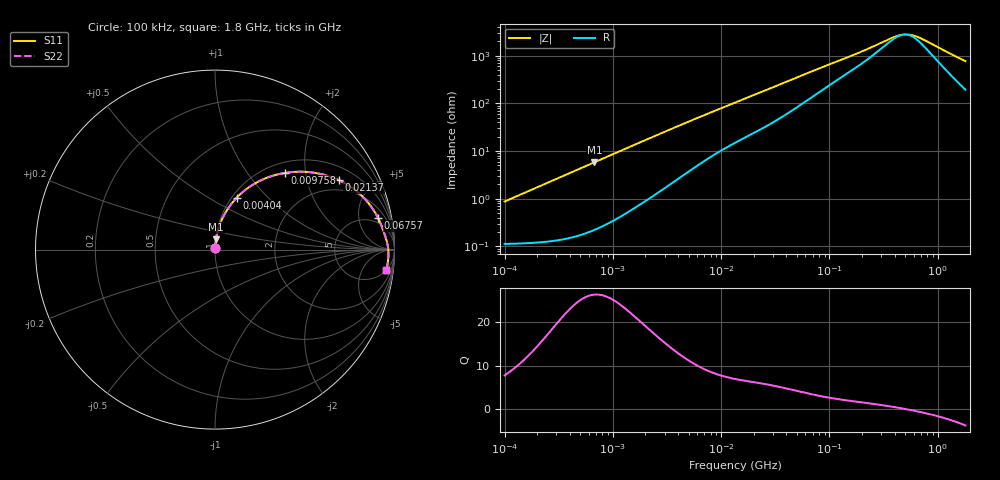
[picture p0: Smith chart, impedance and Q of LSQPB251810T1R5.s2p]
! LSQPB251810T1R5  S-PARAMETER MODEL  ( General Type )
! Model Generated by TAIYO YUDEN Corporation (http://www.ty-top.com)
! Version 2.0
! TAIYO YUDEN Control No. 100810NG22EB-FKC
! Copyright(c) 2009 TAIYO YUDEN CO.,LTD. All Rights Reserved.
! Product Description (link to TY-COMPAS)
! https://ds.yuden.co.jp/TYCOMPAS/or/detail?pn=LSQPB251810T1R5M&u=M
! Products Name : Inductors
! Characteristics :
!  Inductance : 1.5 uH , SRF(min) : 100 MHz , DC Resistance(max) : 0.143 Ohm
!  Rated Current : Saturation :1100 mA , Temp Rise : 1000 mA (40 degC)
!  Case Size : 2.5 x 1.8 / 0.098 x 0.071 [mm/inch] , Thickness : 1.0 / 0.04 [mm/inch]
!  (Conditions: Temperature = 25 degC , DC Bias Current/Voltage = 0A / 0V)
! External Node Assignments :
!  1  o---GGG---o  2
! GND o---------o GND
! Frequency Range : 0.1MHz  -  1800MHz  [ 402 STEP ]
# MHz S RI R 50
! Freq[MHz].  S11 Real  S11 Imag  S21 Real  S21 Imag  S12 Real  S12 Imag  S22 Real  S22 Imag
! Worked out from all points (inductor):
!   401 points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, 100 kHz to 1.8 GHz, reference 50 ohm
!   read as one part in series: L = 1.38 uH near 105 kHz
!   highest Q = 26.4 at 675.7 kHz (marker M1), where L = 1.38 uH
!   self-resonance near 490.3 MHz
!   S11 on the Smith chart (normalised r, x): 100 kHz: 1.00, +0.02; 4.04 MHz: 1.05, +0.67; 9.758 MHz: 1.20, +1.54; 21.37 MHz: 1.52, +3.13; 67.57 MHz: 3.63, +8.90; 1.8 GHz: 5, -15
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0.1  0.0012 0.00865  0.9988 -0.00865  0.9988 -0.00865  0.0012 0.00865
0.516129  0.00374 0.0444  0.9963 -0.0444  0.9963 -0.0444  0.00374 0.0444
0.675738  0.00559 0.0579  0.9944 -0.0579  0.9944 -0.0579  0.00559 0.0579
1.409041  0.0195 0.1179  0.9805 -0.1179  0.9805 -0.1179  0.0195 0.1179
2.66389  0.0601 0.2091  0.9399 -0.2091  0.9399 -0.2091  0.0601 0.2091
4.039851  0.1208 0.289  0.8792 -0.289  0.8792 -0.289  0.1208 0.289
6.126528  0.2245 0.3697  0.7755 -0.3697  0.7755 -0.3697  0.2245 0.3697
9.75753  0.3893 0.4273  0.6107 -0.4273  0.6107 -0.4273  0.3893 0.4273
13.41641  0.5158 0.4324  0.4842 -0.4324  0.4842 -0.4324  0.5158 0.4324
21.36789  0.6882 0.3877  0.3118 -0.3877  0.3118 -0.3877  0.6882 0.3877
27.97575  0.7684 0.341  0.2316 -0.341  0.2316 -0.341  0.7684 0.341
36.62703  0.8296 0.2878  0.1704 -0.2878  0.1704 -0.2878  0.8296 0.2878
67.57036  0.908 0.1769  0.092 -0.1769  0.092 -0.1769  0.908 0.1769
69.24595  0.9098 0.1731  0.0902 -0.1731  0.0902 -0.1731  0.9098 0.1731
184.4683  0.9509 0.0671  0.0491 -0.0671  0.0491 -0.0671  0.9509 0.0671
357.3983  0.9627 0.0209  0.0373 -0.0209  0.0373 -0.0209  0.9627 0.0209
467.921  0.9651 0.00311  0.0349 -0.00311  0.0349 -0.00311  0.9651 0.00311
528.8877  0.9658 -0.00508  0.0342 0.00508  0.0342 0.00508  0.9658 -0.00508
597.7978  0.9662 -0.0135  0.0338 0.0135  0.0338 0.0135  0.9662 -0.0135
727.2099  0.9663 -0.0275  0.0337 0.0275  0.0337 0.0275  0.9663 -0.0275
1341.573  0.9614 -0.0812  0.0386 0.0812  0.0386 0.0812  0.9614 -0.0812
1800  0.9544 -0.1158  0.0456 0.1158  0.0456 0.1158  0.9544 -0.1158
